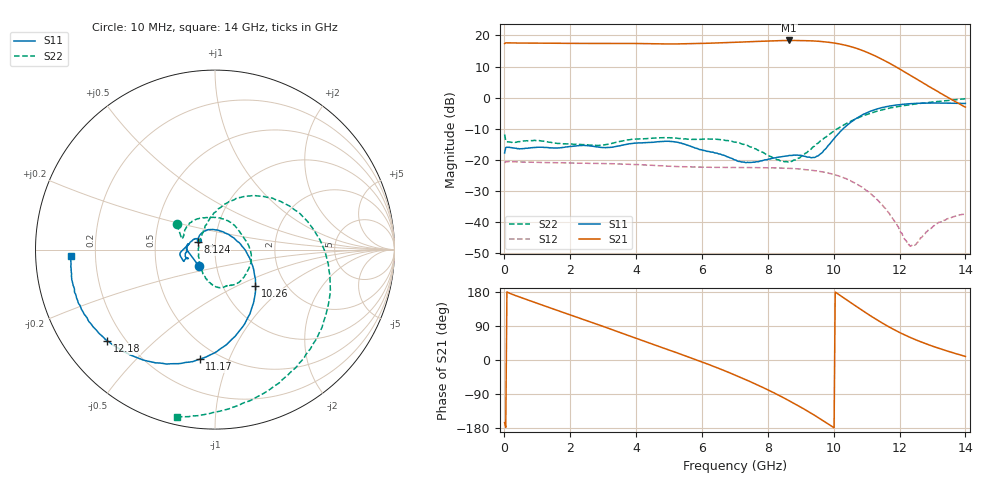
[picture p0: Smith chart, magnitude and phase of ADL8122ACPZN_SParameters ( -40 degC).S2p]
! "Analog Devices, Inc."
! Device:	ADL8122ACPZN
! Description:	"10 kHz to 10 GHz, Wideband, Low Noise Amplifier"
! Conditions:	Vdd = 5.0 V
!		IDQ = 95 mA
!		Pin = -25 dBm
!		Operating Temperature = +25 C (at package bottom)
! Product validation unit SN1 soldered down to Evaluation Board as shown on ADL8122-EVALZ User Guide. Board loss de-embedded from S21 magnitude.  All other RF measurements reference to RF coaxial connector.
! Frequency (GHz)	S11_Mag (dB)	S11_Phase (deg)	S21_Mag (dB)	S21_Phase (deg)	S12_Mag (dB)	S12_Phase (deg)	S22_Mag (dB)	S22_Phase (deg)
#  GHZ  S  DB  R 50
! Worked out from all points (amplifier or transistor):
!   401 points, 10 MHz to 14 GHz, reference 50 ohm
!   highest |S21| = 18.4 dB at 8.649 GHz (marker M1)
!   |S21| within 3 dB of that: start of sweep to 10.82 GHz
!   unconditionally stable (mu >= 1): start of sweep to end of sweep
!   at 2.318 GHz: K = 1.08, MAG = 17.6 dB, |S12| = -21.1 dB
!   at 7.005 GHz: K = 1.11, MAG = 18.1 dB, |S12| = -22.5 dB
!   at 14 GHz: K = 1.16, MAG = 14.8 dB, |S12| = -37.4 dB
!   S11 on the Smith chart (normalised r, x): 10 MHz: 0.82, -0.15; 8.124 GHz: 0.82, +0.07; 10.26 GHz: 1.42, -0.63; 11.17 GHz: 0.40, -0.79; 12.18 GHz: 0.14, -0.36; 14 GHz: 0.11, -0.02
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0.01  -17.84 -134.8  17.38 -165.1  -21.02 15.9  -11.87 146.3
0.1499  -16.02 171.9  17.61 176.6  -20.59 -2.1  -14.32 160.7
0.91935  -16.07 174.8  17.53 152.1  -20.84 -21.7  -13.77 133.8
1.653825  -16.19 -176.3  17.49 129.6  -20.98 -38.8  -14.77 100.8
2.353325  -15.44 -169.1  17.43 108.3  -21.14 -55.4  -15.16 62.2
3.472525  -15.59 -162.9  17.46 73.9  -21.39 -83.9  -14.23 1.5
4.69665  -14.22 -168.2  17.29 35.6  -21.96 -116.5  -12.96 -48.5
5.95575  -16.75 164.4  17.41 -3.5  -22.39 -150.7  -13.47 -73.6
6.480375  -18.01 151.5  17.59 -21.1  -22.47 -165.4  -13.45 -84.5
7.005  -20.07 146.0  17.80 -39.8  -22.52 179.2  -14.33 -97.2
7.529625  -20.84 151.2  18.01 -59.6  -22.57 162.7  -16.08 -113.0
8.1242  -19.59 157.1  18.24 -83.9  -22.65 143.2  -19.15 -141.9
8.648825  -18.64 137.2  18.39 -107.6  -22.81 124.1  -20.55 167.2
9.348325  -19.36 69.6  18.25 -142.1  -23.42 96.2  -16.16 106.2
9.803  -15.87 2.6  17.86 -166.8  -24.23 75.7  -12.40 81.5
10.25768  -10.39 -41.7  17.10 166.9  -25.59 53.2  -9.14 58.6
10.71235  -6.56 -72.7  15.79 139.9  -27.87 29.4  -6.69 33.9
11.16703  -4.20 -97.9  13.87 114.0  -31.34 4.7  -4.88 9.0
11.69165  -2.74 -122.0  11.09 86.8  -37.31 -26.6  -3.40 -18.1
12.1813  -2.09 -139.6  8.11 65.2  -45.90 -81.3  -2.50 -40.3
12.95075  -1.75 -158.8  3.24 38.1  -42.17 163.3  -1.49 -70.2
14  -1.89 -177.5  -3.07 9.4  -37.42 129.4  -0.38 -102.9
